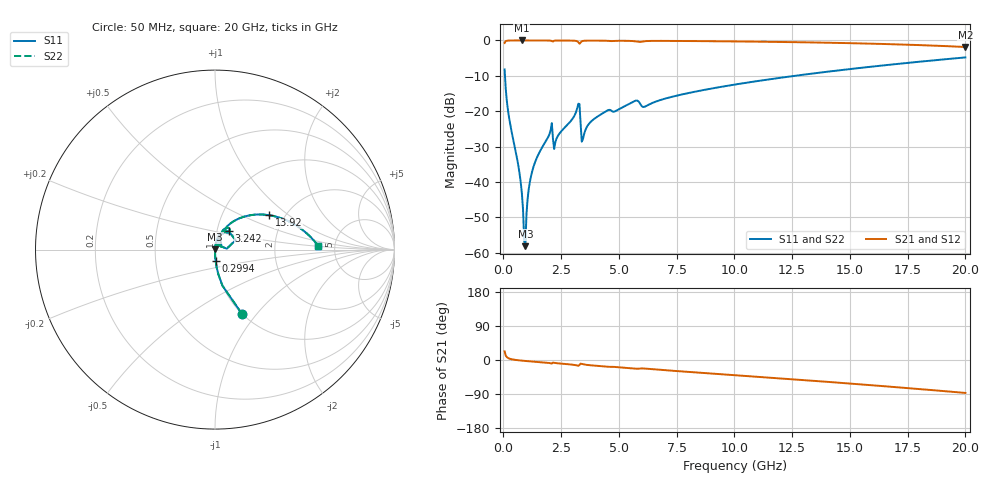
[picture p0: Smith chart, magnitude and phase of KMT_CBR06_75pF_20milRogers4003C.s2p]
! Data measured by Modelithics Inc. support@modelithics.com 813-866-6335
! KEMET CBR0603 75pF, Pad Width= 0.851mm, Pad Length= 0.64mm, Pad Gap= 0.62mm, 20mil Rogers 4003C substrate Data, January 2022
# hz S ma R 50
! 2 Port Network Data from SP1.SP block
! freq  magS11  angS11  magS21  angS21  magS12  angS12  magS22  angS22
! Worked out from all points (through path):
!   401 points, 50 MHz to 20 GHz, reference 50 ohm
!   highest |S21| = 0.00 dB at 798.1 MHz (marker M1); lowest = -1.9 dB at 20 GHz (marker M2)
!   group delay of S21, straight-line fit = 12.2 ps
!   lowest |S11| = -58.2 dB at 947.8 MHz (marker M3), VSWR 1.00, Z = 50.1 + j0.11 ohm
!   |S11| at or under -10 dB: 66.02 MHz to 12.63 GHz (12.56 GHz wide, 198 % of centre)
!   |S22| runs from -58.2 to -4.8 dB; largest |S21 - S12| = 0
!   S11 on the Smith chart (normalised r, x): 50 MHz: 1.00, -0.84; 299.4 MHz: 1.00, -0.13; 3.242 GHz: 1.14, +0.24; 13.92 GHz: 1.66, +0.73; 20 GHz: 3.69, +0.24
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5e7  0.3884 -67.2  0.9212 22.7  0.9212 22.7  0.3884 -67.2
2.99375e8  0.06316 -86.9  0.9977 2.8  0.9977 2.8  0.06316 -86.9
6.485e8  0.01667 -89.3  0.9994 -0.8  0.9994 -0.8  0.01667 -89.3
7.98125e8  0.006846 -87.8  0.9995 -1.7  0.9995 -1.7  0.006846 -87.8
8.48e8  0.00405 -85.2  0.9995 -2.0  0.9995 -2.0  0.00405 -85.2
9.4775e8  0.001231 62.9  0.9995 -2.6  0.9995 -2.6  0.001231 62.9
9.97625e8  0.003542 78.6  0.9994 -2.8  0.9994 -2.8  0.003542 78.6
1.197125e9  0.0122 83.4  0.9993 -3.8  0.9993 -3.8  0.0122 83.4
1.496375e9  0.02385 83.1  0.999 -5.3  0.999 -5.3  0.02385 83.1
1.995125e9  0.04767 79.2  0.9964 -8.0  0.9964 -8.0  0.04767 79.2
2.2445e9  0.03611 76.6  0.9958 -8.0  0.9958 -8.0  0.03611 76.6
3.242e9  0.1274 52.8  0.9454 -15.3  0.9454 -15.3  0.1274 52.8
3.391625e9  0.03704 31.1  0.9718 -10.3  0.9718 -10.3  0.03704 31.1
3.491375e9  0.04734 66.8  0.9894 -11.8  0.9894 -11.8  0.04734 66.8
3.790625e9  0.07125 73.6  0.9944 -14.0  0.9944 -14.0  0.07125 73.6
4.488875e9  0.1017 68.8  0.9883 -17.6  0.9883 -17.6  0.1017 68.8
6.73325e9  0.1415 62.6  0.9857 -25.8  0.9857 -25.8  0.1415 62.6
1.0025e10  0.2379 49.6  0.9687 -39.9  0.9687 -39.9  0.2379 49.6
1.336662e10  0.3398 34.9  0.9372 -54.6  0.9372 -54.6  0.3398 34.9
1.391525e10  0.3575 32.4  0.9304 -57.1  0.9304 -57.1  0.3575 32.4
1.670825e10  0.453 19.2  0.8864 -70.3  0.8864 -70.3  0.453 19.2
2e10  0.5753 2.1  0.8075 -86.9  0.8075 -86.9  0.5753 2.1
